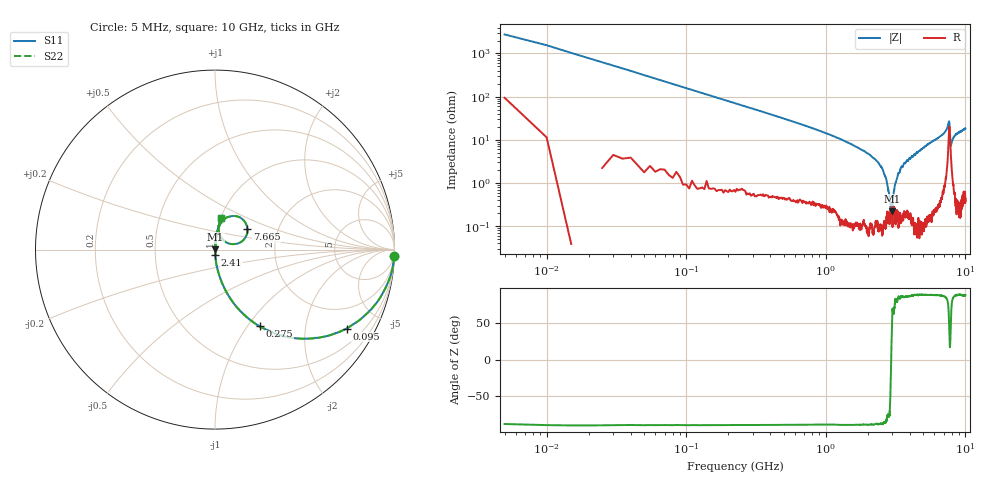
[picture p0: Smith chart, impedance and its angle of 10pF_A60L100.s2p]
! Amotech Co.,Ltd.
! http://www.amotech.co.kr/
! Part Number: A60L100
! These Parameters are Measured in Series Mode Connection
! Operation Temp=25[degC], DC Bias Voltage=0[V]
! Freq. Start=5[MHz] Stop=10[GHz], 2000[Steps]
! Date: Monday, July 14, 2020, 09:35:43
# GHZ S RI R 50.000000
!Freq.(Hz) S11(Real) S11(Imag) S21(Real) S21(Imag) S12(Real) S12(Imag) S22(Real) S22(Imag)
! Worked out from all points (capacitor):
!   2000 points, 5 MHz to 10 GHz, reference 50 ohm
!   read as one part in series: C = 10.1 pF near 55 MHz
!   lowest |Z| = 219 mohm at 2.97 GHz (marker M1)
!   series resonance near 2.939 GHz, so ESL is about 290 pH
!   S11 on the Smith chart (normalised r, x): 5 MHz: 3, -55; 95 MHz: 1.02, -3.32; 275 MHz: 1.01, -1.14; 2.41 GHz: 1.00, -0.06; 7.665 GHz: 1.39, +0.33; 10 GHz: 1.01, +0.37
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0.005  0.9975 -0.0361  0.00254 0.0361  0.00254 0.0361  0.9975 -0.0361
0.065  0.8533 -0.3496  0.1467 0.3496  0.1467 0.3496  0.8533 -0.3496
0.095  0.7328 -0.4398  0.2672 0.4398  0.2672 0.4398  0.7328 -0.4398
0.165  0.4786 -0.4962  0.5214 0.4962  0.5214 0.4962  0.4786 -0.4962
0.275  0.249 -0.4274  0.751 0.4274  0.751 0.4274  0.249 -0.4274
0.635  0.0581 -0.2263  0.9419 0.2263  0.9419 0.2263  0.0581 -0.2263
1.675  0.0057 -0.0668  0.9943 0.0668  0.9943 0.0668  0.0057 -0.0668
2.41  0.00167 -0.0276  0.9983 0.0276  0.9983 0.0276  0.00167 -0.0276
2.7  0.00115 -0.0129  0.9989 0.0129  0.9989 0.0129  0.00115 -0.0129
2.925  0.00271 -0.00104  0.9973 0.00104  0.9973 0.00104  0.00271 -0.00104
2.97  0.00183 0.00121  0.9982 -0.00121  0.9982 -0.00121  0.00183 0.00121
3.125  0.00201 0.00834  0.998 -0.00834  0.998 -0.00834  0.00201 0.00834
3.34  0.00145 0.0172  0.9985 -0.0172  0.9985 -0.0172  0.00145 0.0172
3.805  0.00318 0.0327  0.9968 -0.0327  0.9968 -0.0327  0.00318 0.0327
5.005  0.00512 0.0653  0.9949 -0.0653  0.9949 -0.0653  0.00512 0.0653
6.67  0.0185 0.1197  0.9815 -0.1197  0.9815 -0.1197  0.0185 0.1197
7.38  0.0512 0.1681  0.9488 -0.1681  0.9488 -0.1681  0.0512 0.1681
7.665  0.1805 0.1134  0.8195 -0.1134  0.8195 -0.1134  0.1805 0.1134
7.805  0.0731 0.0354  0.9269 -0.0354  0.9269 -0.0354  0.0731 0.0354
7.86  0.0482 0.0505  0.9518 -0.0505  0.9518 -0.0505  0.0482 0.0505
8.335  0.0196 0.1175  0.9804 -0.1175  0.9804 -0.1175  0.0196 0.1175
10  0.036 0.1761  0.964 -0.1761  0.964 -0.1761  0.036 0.1761
